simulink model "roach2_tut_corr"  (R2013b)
settings: Solver=VariableStepDiscrete  SolverMode=SingleTasking  StartTime=0.0  StopTime=100  RelTol=1e-3
undefined symbols (not defined in the file): add_latency, addr_width, Bit, bitfield, BitWidth, bram_latency, burst_size, casper_library_scopes, conv_latency, data_width, DelayLen, fan_latency, FFTSize, FFTStage, getfield, increment, led, Location, Lower, mult_latency, mux_latency, n_bits, n_bits_data, n_inputs, n_streams, n_taps, neg_latency, negate_latency, nsamples, pfb_size, pulse_len, reset_period, ROACH, ROACH2, snapshot, sx475t, sync_period, sync_period_bits, Upper, UseCounter, Width
libraries: xbsIndex_r4 x24444, casper_library_misc x73, xbsReplacements_r4 x34, casper_library_delays x14, xps_library x7
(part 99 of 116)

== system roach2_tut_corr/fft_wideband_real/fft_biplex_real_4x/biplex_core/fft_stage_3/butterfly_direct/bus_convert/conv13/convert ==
  note: (ones_bit & 1) -> round-to-even (ones_bit ^ 1) -> round-to-odd (sign_bit & 1)-> round-to-zero (sign_bit ^ 1) -> round-to-inf (X ~| 1) -> round half down (X | 1) -> round half up
  in : Inport
  Concat : xbsIndex_r4/Concat  num_inputs=2  dbl_ovrd=off  block_type=concat
  Constant : xbsIndex_r4/Constant  const=1  gui_display_data_type=Fixed-point  arith_type=Unsigned  n_bits=1  bin_pt=0  preci_type=Single  exp_width=8  frac_width=24  explicit_period=off  period=1  equ=P=C  opselect=C  inp2=PCIN>>17  opr=+  inp1=P  carry=CIN  dbl_ovrd=off  block_type=constant
  Reinterpret : xbsIndex_r4/Reinterpret  force_arith_type=on  arith_type=Unsigned  force_bin_pt=on  bin_pt=0  block_type=reinterpret
  adder : xbsIndex_r4/AddSub  mode=Addition  use_carryin=off  use_carryout=off  en=off  latency=1  precision=User Defined  arith_type="Signed  (2's comp)"  n_bits=18  bin_pt=17  quantization=Truncate  overflow=Wrap  dbl_ovrd=off  use_behavioral_HDL=off  hw_selection=Fabric  pipelined=on  use_rpm=on  block_type=addsub
  almost_half : xbsIndex_r4/Constant  const=1  gui_display_data_type=Fixed-point  arith_type=Unsigned  n_bits=19  bin_pt=0  preci_type=Single  exp_width=8  frac_width=24  explicit_period=off  period=1  equ=P=C  opselect=C  inp2=PCIN>>17  opr=+  inp1=P  carry=CIN  dbl_ovrd=off  block_type=constant
  bit : xbsIndex_r4/Slice  nbits=1  boolean_output=off  mode=Lower Bit Location + Width  bit1=0  base1=MSB of Input  bit0=1  base0=LSB of Input  dbl_ovrd=off  block_type=slice
  force1 : xbsIndex_r4/Reinterpret  force_arith_type=on  arith_type="Signed  (2's comp)"  force_bin_pt=on  bin_pt=19  block_type=reinterpret
  force2 : xbsIndex_r4/Reinterpret  force_arith_type=off  arith_type="Signed  (2's comp)"  force_bin_pt=on  bin_pt=19  block_type=reinterpret
  tweak_op : xbsIndex_r4/Logical  logical_function=AND  inputs=2  en=off  latency=0  precision=Full  arith_type=Unsigned  n_bits=8  bin_pt=2  align_bp=on  dbl_ovrd=off  block_type=logical
  out : Outport
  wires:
  tweak_op/1 -> Concat/2
  Constant/1 -> tweak_op/2
  bit/1 -> tweak_op/1
  almost_half/1 -> force2/1
  in/1 -> Reinterpret/1, bit/1
  Concat/1 -> force1/1
  Reinterpret/1 -> Concat/1
  force1/1 -> adder/1
  force2/1 -> adder/2
  adder/1 -> out/1

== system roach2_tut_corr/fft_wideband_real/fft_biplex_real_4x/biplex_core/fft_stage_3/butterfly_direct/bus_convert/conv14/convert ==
  note: (ones_bit & 1) -> round-to-even (ones_bit ^ 1) -> round-to-odd (sign_bit & 1)-> round-to-zero (sign_bit ^ 1) -> round-to-inf (X ~| 1) -> round half down (X | 1) -> round half up
  in : Inport
  Concat : xbsIndex_r4/Concat  num_inputs=2  dbl_ovrd=off  block_type=concat
  Constant : xbsIndex_r4/Constant  const=1  gui_display_data_type=Fixed-point  arith_type=Unsigned  n_bits=1  bin_pt=0  preci_type=Single  exp_width=8  frac_width=24  explicit_period=off  period=1  equ=P=C  opselect=C  inp2=PCIN>>17  opr=+  inp1=P  carry=CIN  dbl_ovrd=off  block_type=constant
  Reinterpret : xbsIndex_r4/Reinterpret  force_arith_type=on  arith_type=Unsigned  force_bin_pt=on  bin_pt=0  block_type=reinterpret
  adder : xbsIndex_r4/AddSub  mode=Addition  use_carryin=off  use_carryout=off  en=off  latency=1  precision=User Defined  arith_type="Signed  (2's comp)"  n_bits=18  bin_pt=17  quantization=Truncate  overflow=Wrap  dbl_ovrd=off  use_behavioral_HDL=off  hw_selection=Fabric  pipelined=on  use_rpm=on  block_type=addsub
  almost_half : xbsIndex_r4/Constant  const=1  gui_display_data_type=Fixed-point  arith_type=Unsigned  n_bits=19  bin_pt=0  preci_type=Single  exp_width=8  frac_width=24  explicit_period=off  period=1  equ=P=C  opselect=C  inp2=PCIN>>17  opr=+  inp1=P  carry=CIN  dbl_ovrd=off  block_type=constant
  bit : xbsIndex_r4/Slice  nbits=1  boolean_output=off  mode=Lower Bit Location + Width  bit1=0  base1=MSB of Input  bit0=1  base0=LSB of Input  dbl_ovrd=off  block_type=slice
  force1 : xbsIndex_r4/Reinterpret  force_arith_type=on  arith_type="Signed  (2's comp)"  force_bin_pt=on  bin_pt=19  block_type=reinterpret
  force2 : xbsIndex_r4/Reinterpret  force_arith_type=off  arith_type="Signed  (2's comp)"  force_bin_pt=on  bin_pt=19  block_type=reinterpret
  tweak_op : xbsIndex_r4/Logical  logical_function=AND  inputs=2  en=off  latency=0  precision=Full  arith_type=Unsigned  n_bits=8  bin_pt=2  align_bp=on  dbl_ovrd=off  block_type=logical
  out : Outport
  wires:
  tweak_op/1 -> Concat/2
  Constant/1 -> tweak_op/2
  bit/1 -> tweak_op/1
  almost_half/1 -> force2/1
  in/1 -> Reinterpret/1, bit/1
  Concat/1 -> force1/1
  Reinterpret/1 -> Concat/1
  force1/1 -> adder/1
  force2/1 -> adder/2
  adder/1 -> out/1

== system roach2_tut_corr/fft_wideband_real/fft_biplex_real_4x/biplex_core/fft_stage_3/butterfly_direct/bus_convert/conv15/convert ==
  note: (ones_bit & 1) -> round-to-even (ones_bit ^ 1) -> round-to-odd (sign_bit & 1)-> round-to-zero (sign_bit ^ 1) -> round-to-inf (X ~| 1) -> round half down (X | 1) -> round half up
  in : Inport
  Concat : xbsIndex_r4/Concat  num_inputs=2  dbl_ovrd=off  block_type=concat
  Constant : xbsIndex_r4/Constant  const=1  gui_display_data_type=Fixed-point  arith_type=Unsigned  n_bits=1  bin_pt=0  preci_type=Single  exp_width=8  frac_width=24  explicit_period=off  period=1  equ=P=C  opselect=C  inp2=PCIN>>17  opr=+  inp1=P  carry=CIN  dbl_ovrd=off  block_type=constant
  Reinterpret : xbsIndex_r4/Reinterpret  force_arith_type=on  arith_type=Unsigned  force_bin_pt=on  bin_pt=0  block_type=reinterpret
  adder : xbsIndex_r4/AddSub  mode=Addition  use_carryin=off  use_carryout=off  en=off  latency=1  precision=User Defined  arith_type="Signed  (2's comp)"  n_bits=18  bin_pt=17  quantization=Truncate  overflow=Wrap  dbl_ovrd=off  use_behavioral_HDL=off  hw_selection=Fabric  pipelined=on  use_rpm=on  block_type=addsub
  almost_half : xbsIndex_r4/Constant  const=1  gui_display_data_type=Fixed-point  arith_type=Unsigned  n_bits=19  bin_pt=0  preci_type=Single  exp_width=8  frac_width=24  explicit_period=off  period=1  equ=P=C  opselect=C  inp2=PCIN>>17  opr=+  inp1=P  carry=CIN  dbl_ovrd=off  block_type=constant
  bit : xbsIndex_r4/Slice  nbits=1  boolean_output=off  mode=Lower Bit Location + Width  bit1=0  base1=MSB of Input  bit0=1  base0=LSB of Input  dbl_ovrd=off  block_type=slice
  force1 : xbsIndex_r4/Reinterpret  force_arith_type=on  arith_type="Signed  (2's comp)"  force_bin_pt=on  bin_pt=19  block_type=reinterpret
  force2 : xbsIndex_r4/Reinterpret  force_arith_type=off  arith_type="Signed  (2's comp)"  force_bin_pt=on  bin_pt=19  block_type=reinterpret
  tweak_op : xbsIndex_r4/Logical  logical_function=AND  inputs=2  en=off  latency=0  precision=Full  arith_type=Unsigned  n_bits=8  bin_pt=2  align_bp=on  dbl_ovrd=off  block_type=logical
  out : Outport
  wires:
  tweak_op/1 -> Concat/2
  Constant/1 -> tweak_op/2
  bit/1 -> tweak_op/1
  almost_half/1 -> force2/1
  in/1 -> Reinterpret/1, bit/1
  Concat/1 -> force1/1
  Reinterpret/1 -> Concat/1
  force1/1 -> adder/1
  force2/1 -> adder/2
  adder/1 -> out/1

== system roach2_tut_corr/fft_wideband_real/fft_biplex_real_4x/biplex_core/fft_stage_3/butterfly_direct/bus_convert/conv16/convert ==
  note: (ones_bit & 1) -> round-to-even (ones_bit ^ 1) -> round-to-odd (sign_bit & 1)-> round-to-zero (sign_bit ^ 1) -> round-to-inf (X ~| 1) -> round half down (X | 1) -> round half up
  in : Inport
  Concat : xbsIndex_r4/Concat  num_inputs=2  dbl_ovrd=off  block_type=concat
  Constant : xbsIndex_r4/Constant  const=1  gui_display_data_type=Fixed-point  arith_type=Unsigned  n_bits=1  bin_pt=0  preci_type=Single  exp_width=8  frac_width=24  explicit_period=off  period=1  equ=P=C  opselect=C  inp2=PCIN>>17  opr=+  inp1=P  carry=CIN  dbl_ovrd=off  block_type=constant
  Reinterpret : xbsIndex_r4/Reinterpret  force_arith_type=on  arith_type=Unsigned  force_bin_pt=on  bin_pt=0  block_type=reinterpret
  adder : xbsIndex_r4/AddSub  mode=Addition  use_carryin=off  use_carryout=off  en=off  latency=1  precision=User Defined  arith_type="Signed  (2's comp)"  n_bits=18  bin_pt=17  quantization=Truncate  overflow=Wrap  dbl_ovrd=off  use_behavioral_HDL=off  hw_selection=Fabric  pipelined=on  use_rpm=on  block_type=addsub
  almost_half : xbsIndex_r4/Constant  const=1  gui_display_data_type=Fixed-point  arith_type=Unsigned  n_bits=19  bin_pt=0  preci_type=Single  exp_width=8  frac_width=24  explicit_period=off  period=1  equ=P=C  opselect=C  inp2=PCIN>>17  opr=+  inp1=P  carry=CIN  dbl_ovrd=off  block_type=constant
  bit : xbsIndex_r4/Slice  nbits=1  boolean_output=off  mode=Lower Bit Location + Width  bit1=0  base1=MSB of Input  bit0=1  base0=LSB of Input  dbl_ovrd=off  block_type=slice
  force1 : xbsIndex_r4/Reinterpret  force_arith_type=on  arith_type="Signed  (2's comp)"  force_bin_pt=on  bin_pt=19  block_type=reinterpret
  force2 : xbsIndex_r4/Reinterpret  force_arith_type=off  arith_type="Signed  (2's comp)"  force_bin_pt=on  bin_pt=19  block_type=reinterpret
  tweak_op : xbsIndex_r4/Logical  logical_function=AND  inputs=2  en=off  latency=0  precision=Full  arith_type=Unsigned  n_bits=8  bin_pt=2  align_bp=on  dbl_ovrd=off  block_type=logical
  out : Outport
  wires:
  tweak_op/1 -> Concat/2
  Constant/1 -> tweak_op/2
  bit/1 -> tweak_op/1
  almost_half/1 -> force2/1
  in/1 -> Reinterpret/1, bit/1
  Concat/1 -> force1/1
  Reinterpret/1 -> Concat/1
  force1/1 -> adder/1
  force2/1 -> adder/2
  adder/1 -> out/1

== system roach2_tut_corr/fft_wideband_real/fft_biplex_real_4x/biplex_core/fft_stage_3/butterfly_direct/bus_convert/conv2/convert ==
  note: (ones_bit & 1) -> round-to-even (ones_bit ^ 1) -> round-to-odd (sign_bit & 1)-> round-to-zero (sign_bit ^ 1) -> round-to-inf (X ~| 1) -> round half down (X | 1) -> round half up
  in : Inport
  Concat : xbsIndex_r4/Concat  num_inputs=2  dbl_ovrd=off  block_type=concat
  Constant : xbsIndex_r4/Constant  const=1  gui_display_data_type=Fixed-point  arith_type=Unsigned  n_bits=1  bin_pt=0  preci_type=Single  exp_width=8  frac_width=24  explicit_period=off  period=1  equ=P=C  opselect=C  inp2=PCIN>>17  opr=+  inp1=P  carry=CIN  dbl_ovrd=off  block_type=constant
  Reinterpret : xbsIndex_r4/Reinterpret  force_arith_type=on  arith_type=Unsigned  force_bin_pt=on  bin_pt=0  block_type=reinterpret
  adder : xbsIndex_r4/AddSub  mode=Addition  use_carryin=off  use_carryout=off  en=off  latency=1  precision=User Defined  arith_type="Signed  (2's comp)"  n_bits=18  bin_pt=17  quantization=Truncate  overflow=Wrap  dbl_ovrd=off  use_behavioral_HDL=off  hw_selection=Fabric  pipelined=on  use_rpm=on  block_type=addsub
  almost_half : xbsIndex_r4/Constant  const=1  gui_display_data_type=Fixed-point  arith_type=Unsigned  n_bits=19  bin_pt=0  preci_type=Single  exp_width=8  frac_width=24  explicit_period=off  period=1  equ=P=C  opselect=C  inp2=PCIN>>17  opr=+  inp1=P  carry=CIN  dbl_ovrd=off  block_type=constant
  bit : xbsIndex_r4/Slice  nbits=1  boolean_output=off  mode=Lower Bit Location + Width  bit1=0  base1=MSB of Input  bit0=1  base0=LSB of Input  dbl_ovrd=off  block_type=slice
  force1 : xbsIndex_r4/Reinterpret  force_arith_type=on  arith_type="Signed  (2's comp)"  force_bin_pt=on  bin_pt=19  block_type=reinterpret
  force2 : xbsIndex_r4/Reinterpret  force_arith_type=off  arith_type="Signed  (2's comp)"  force_bin_pt=on  bin_pt=19  block_type=reinterpret
  tweak_op : xbsIndex_r4/Logical  logical_function=AND  inputs=2  en=off  latency=0  precision=Full  arith_type=Unsigned  n_bits=8  bin_pt=2  align_bp=on  dbl_ovrd=off  block_type=logical
  out : Outport
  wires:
  tweak_op/1 -> Concat/2
  Constant/1 -> tweak_op/2
  bit/1 -> tweak_op/1
  almost_half/1 -> force2/1
  in/1 -> Reinterpret/1, bit/1
  Concat/1 -> force1/1
  Reinterpret/1 -> Concat/1
  force1/1 -> adder/1
  force2/1 -> adder/2
  adder/1 -> out/1

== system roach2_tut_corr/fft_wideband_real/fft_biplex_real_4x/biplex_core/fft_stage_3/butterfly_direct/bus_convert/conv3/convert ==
  note: (ones_bit & 1) -> round-to-even (ones_bit ^ 1) -> round-to-odd (sign_bit & 1)-> round-to-zero (sign_bit ^ 1) -> round-to-inf (X ~| 1) -> round half down (X | 1) -> round half up
  in : Inport
  Concat : xbsIndex_r4/Concat  num_inputs=2  dbl_ovrd=off  block_type=concat
  Constant : xbsIndex_r4/Constant  const=1  gui_display_data_type=Fixed-point  arith_type=Unsigned  n_bits=1  bin_pt=0  preci_type=Single  exp_width=8  frac_width=24  explicit_period=off  period=1  equ=P=C  opselect=C  inp2=PCIN>>17  opr=+  inp1=P  carry=CIN  dbl_ovrd=off  block_type=constant
  Reinterpret : xbsIndex_r4/Reinterpret  force_arith_type=on  arith_type=Unsigned  force_bin_pt=on  bin_pt=0  block_type=reinterpret
  adder : xbsIndex_r4/AddSub  mode=Addition  use_carryin=off  use_carryout=off  en=off  latency=1  precision=User Defined  arith_type="Signed  (2's comp)"  n_bits=18  bin_pt=17  quantization=Truncate  overflow=Wrap  dbl_ovrd=off  use_behavioral_HDL=off  hw_selection=Fabric  pipelined=on  use_rpm=on  block_type=addsub
  almost_half : xbsIndex_r4/Constant  const=1  gui_display_data_type=Fixed-point  arith_type=Unsigned  n_bits=19  bin_pt=0  preci_type=Single  exp_width=8  frac_width=24  explicit_period=off  period=1  equ=P=C  opselect=C  inp2=PCIN>>17  opr=+  inp1=P  carry=CIN  dbl_ovrd=off  block_type=constant
  bit : xbsIndex_r4/Slice  nbits=1  boolean_output=off  mode=Lower Bit Location + Width  bit1=0  base1=MSB of Input  bit0=1  base0=LSB of Input  dbl_ovrd=off  block_type=slice
  force1 : xbsIndex_r4/Reinterpret  force_arith_type=on  arith_type="Signed  (2's comp)"  force_bin_pt=on  bin_pt=19  block_type=reinterpret
  force2 : xbsIndex_r4/Reinterpret  force_arith_type=off  arith_type="Signed  (2's comp)"  force_bin_pt=on  bin_pt=19  block_type=reinterpret
  tweak_op : xbsIndex_r4/Logical  logical_function=AND  inputs=2  en=off  latency=0  precision=Full  arith_type=Unsigned  n_bits=8  bin_pt=2  align_bp=on  dbl_ovrd=off  block_type=logical
  out : Outport
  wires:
  tweak_op/1 -> Concat/2
  Constant/1 -> tweak_op/2
  bit/1 -> tweak_op/1
  almost_half/1 -> force2/1
  in/1 -> Reinterpret/1, bit/1
  Concat/1 -> force1/1
  Reinterpret/1 -> Concat/1
  force1/1 -> adder/1
  force2/1 -> adder/2
  adder/1 -> out/1

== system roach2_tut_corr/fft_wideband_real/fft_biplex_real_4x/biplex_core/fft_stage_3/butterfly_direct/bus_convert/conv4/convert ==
  note: (ones_bit & 1) -> round-to-even (ones_bit ^ 1) -> round-to-odd (sign_bit & 1)-> round-to-zero (sign_bit ^ 1) -> round-to-inf (X ~| 1) -> round half down (X | 1) -> round half up
  in : Inport
  Concat : xbsIndex_r4/Concat  num_inputs=2  dbl_ovrd=off  block_type=concat
  Constant : xbsIndex_r4/Constant  const=1  gui_display_data_type=Fixed-point  arith_type=Unsigned  n_bits=1  bin_pt=0  preci_type=Single  exp_width=8  frac_width=24  explicit_period=off  period=1  equ=P=C  opselect=C  inp2=PCIN>>17  opr=+  inp1=P  carry=CIN  dbl_ovrd=off  block_type=constant
  Reinterpret : xbsIndex_r4/Reinterpret  force_arith_type=on  arith_type=Unsigned  force_bin_pt=on  bin_pt=0  block_type=reinterpret
  adder : xbsIndex_r4/AddSub  mode=Addition  use_carryin=off  use_carryout=off  en=off  latency=1  precision=User Defined  arith_type="Signed  (2's comp)"  n_bits=18  bin_pt=17  quantization=Truncate  overflow=Wrap  dbl_ovrd=off  use_behavioral_HDL=off  hw_selection=Fabric  pipelined=on  use_rpm=on  block_type=addsub
  almost_half : xbsIndex_r4/Constant  const=1  gui_display_data_type=Fixed-point  arith_type=Unsigned  n_bits=19  bin_pt=0  preci_type=Single  exp_width=8  frac_width=24  explicit_period=off  period=1  equ=P=C  opselect=C  inp2=PCIN>>17  opr=+  inp1=P  carry=CIN  dbl_ovrd=off  block_type=constant
  bit : xbsIndex_r4/Slice  nbits=1  boolean_output=off  mode=Lower Bit Location + Width  bit1=0  base1=MSB of Input  bit0=1  base0=LSB of Input  dbl_ovrd=off  block_type=slice
  force1 : xbsIndex_r4/Reinterpret  force_arith_type=on  arith_type="Signed  (2's comp)"  force_bin_pt=on  bin_pt=19  block_type=reinterpret
  force2 : xbsIndex_r4/Reinterpret  force_arith_type=off  arith_type="Signed  (2's comp)"  force_bin_pt=on  bin_pt=19  block_type=reinterpret
  tweak_op : xbsIndex_r4/Logical  logical_function=AND  inputs=2  en=off  latency=0  precision=Full  arith_type=Unsigned  n_bits=8  bin_pt=2  align_bp=on  dbl_ovrd=off  block_type=logical
  out : Outport
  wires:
  tweak_op/1 -> Concat/2
  Constant/1 -> tweak_op/2
  bit/1 -> tweak_op/1
  almost_half/1 -> force2/1
  in/1 -> Reinterpret/1, bit/1
  Concat/1 -> force1/1
  Reinterpret/1 -> Concat/1
  force1/1 -> adder/1
  force2/1 -> adder/2
  adder/1 -> out/1

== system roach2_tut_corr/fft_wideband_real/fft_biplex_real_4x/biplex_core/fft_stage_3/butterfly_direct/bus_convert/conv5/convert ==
  note: (ones_bit & 1) -> round-to-even (ones_bit ^ 1) -> round-to-odd (sign_bit & 1)-> round-to-zero (sign_bit ^ 1) -> round-to-inf (X ~| 1) -> round half down (X | 1) -> round half up
  in : Inport
  Concat : xbsIndex_r4/Concat  num_inputs=2  dbl_ovrd=off  block_type=concat
  Constant : xbsIndex_r4/Constant  const=1  gui_display_data_type=Fixed-point  arith_type=Unsigned  n_bits=1  bin_pt=0  preci_type=Single  exp_width=8  frac_width=24  explicit_period=off  period=1  equ=P=C  opselect=C  inp2=PCIN>>17  opr=+  inp1=P  carry=CIN  dbl_ovrd=off  block_type=constant
  Reinterpret : xbsIndex_r4/Reinterpret  force_arith_type=on  arith_type=Unsigned  force_bin_pt=on  bin_pt=0  block_type=reinterpret
  adder : xbsIndex_r4/AddSub  mode=Addition  use_carryin=off  use_carryout=off  en=off  latency=1  precision=User Defined  arith_type="Signed  (2's comp)"  n_bits=18  bin_pt=17  quantization=Truncate  overflow=Wrap  dbl_ovrd=off  use_behavioral_HDL=off  hw_selection=Fabric  pipelined=on  use_rpm=on  block_type=addsub
  almost_half : xbsIndex_r4/Constant  const=1  gui_display_data_type=Fixed-point  arith_type=Unsigned  n_bits=19  bin_pt=0  preci_type=Single  exp_width=8  frac_width=24  explicit_period=off  period=1  equ=P=C  opselect=C  inp2=PCIN>>17  opr=+  inp1=P  carry=CIN  dbl_ovrd=off  block_type=constant
  bit : xbsIndex_r4/Slice  nbits=1  boolean_output=off  mode=Lower Bit Location + Width  bit1=0  base1=MSB of Input  bit0=1  base0=LSB of Input  dbl_ovrd=off  block_type=slice
  force1 : xbsIndex_r4/Reinterpret  force_arith_type=on  arith_type="Signed  (2's comp)"  force_bin_pt=on  bin_pt=19  block_type=reinterpret
  force2 : xbsIndex_r4/Reinterpret  force_arith_type=off  arith_type="Signed  (2's comp)"  force_bin_pt=on  bin_pt=19  block_type=reinterpret
  tweak_op : xbsIndex_r4/Logical  logical_function=AND  inputs=2  en=off  latency=0  precision=Full  arith_type=Unsigned  n_bits=8  bin_pt=2  align_bp=on  dbl_ovrd=off  block_type=logical
  out : Outport
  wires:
  tweak_op/1 -> Concat/2
  Constant/1 -> tweak_op/2
  bit/1 -> tweak_op/1
  almost_half/1 -> force2/1
  in/1 -> Reinterpret/1, bit/1
  Concat/1 -> force1/1
  Reinterpret/1 -> Concat/1
  force1/1 -> adder/1
  force2/1 -> adder/2
  adder/1 -> out/1

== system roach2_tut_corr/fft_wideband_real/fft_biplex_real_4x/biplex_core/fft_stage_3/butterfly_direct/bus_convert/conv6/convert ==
  note: (ones_bit & 1) -> round-to-even (ones_bit ^ 1) -> round-to-odd (sign_bit & 1)-> round-to-zero (sign_bit ^ 1) -> round-to-inf (X ~| 1) -> round half down (X | 1) -> round half up
  in : Inport
  Concat : xbsIndex_r4/Concat  num_inputs=2  dbl_ovrd=off  block_type=concat
  Constant : xbsIndex_r4/Constant  const=1  gui_display_data_type=Fixed-point  arith_type=Unsigned  n_bits=1  bin_pt=0  preci_type=Single  exp_width=8  frac_width=24  explicit_period=off  period=1  equ=P=C  opselect=C  inp2=PCIN>>17  opr=+  inp1=P  carry=CIN  dbl_ovrd=off  block_type=constant
  Reinterpret : xbsIndex_r4/Reinterpret  force_arith_type=on  arith_type=Unsigned  force_bin_pt=on  bin_pt=0  block_type=reinterpret
  adder : xbsIndex_r4/AddSub  mode=Addition  use_carryin=off  use_carryout=off  en=off  latency=1  precision=User Defined  arith_type="Signed  (2's comp)"  n_bits=18  bin_pt=17  quantization=Truncate  overflow=Wrap  dbl_ovrd=off  use_behavioral_HDL=off  hw_selection=Fabric  pipelined=on  use_rpm=on  block_type=addsub
  almost_half : xbsIndex_r4/Constant  const=1  gui_display_data_type=Fixed-point  arith_type=Unsigned  n_bits=19  bin_pt=0  preci_type=Single  exp_width=8  frac_width=24  explicit_period=off  period=1  equ=P=C  opselect=C  inp2=PCIN>>17  opr=+  inp1=P  carry=CIN  dbl_ovrd=off  block_type=constant
  bit : xbsIndex_r4/Slice  nbits=1  boolean_output=off  mode=Lower Bit Location + Width  bit1=0  base1=MSB of Input  bit0=1  base0=LSB of Input  dbl_ovrd=off  block_type=slice
  force1 : xbsIndex_r4/Reinterpret  force_arith_type=on  arith_type="Signed  (2's comp)"  force_bin_pt=on  bin_pt=19  block_type=reinterpret
  force2 : xbsIndex_r4/Reinterpret  force_arith_type=off  arith_type="Signed  (2's comp)"  force_bin_pt=on  bin_pt=19  block_type=reinterpret
  tweak_op : xbsIndex_r4/Logical  logical_function=AND  inputs=2  en=off  latency=0  precision=Full  arith_type=Unsigned  n_bits=8  bin_pt=2  align_bp=on  dbl_ovrd=off  block_type=logical
  out : Outport
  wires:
  tweak_op/1 -> Concat/2
  Constant/1 -> tweak_op/2
  bit/1 -> tweak_op/1
  almost_half/1 -> force2/1
  in/1 -> Reinterpret/1, bit/1
  Concat/1 -> force1/1
  Reinterpret/1 -> Concat/1
  force1/1 -> adder/1
  force2/1 -> adder/2
  adder/1 -> out/1

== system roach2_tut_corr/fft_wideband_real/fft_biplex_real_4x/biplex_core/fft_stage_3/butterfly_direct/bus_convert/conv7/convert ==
  note: (ones_bit & 1) -> round-to-even (ones_bit ^ 1) -> round-to-odd (sign_bit & 1)-> round-to-zero (sign_bit ^ 1) -> round-to-inf (X ~| 1) -> round half down (X | 1) -> round half up
  in : Inport
  Concat : xbsIndex_r4/Concat  num_inputs=2  dbl_ovrd=off  block_type=concat
  Constant : xbsIndex_r4/Constant  const=1  gui_display_data_type=Fixed-point  arith_type=Unsigned  n_bits=1  bin_pt=0  preci_type=Single  exp_width=8  frac_width=24  explicit_period=off  period=1  equ=P=C  opselect=C  inp2=PCIN>>17  opr=+  inp1=P  carry=CIN  dbl_ovrd=off  block_type=constant
  Reinterpret : xbsIndex_r4/Reinterpret  force_arith_type=on  arith_type=Unsigned  force_bin_pt=on  bin_pt=0  block_type=reinterpret
  adder : xbsIndex_r4/AddSub  mode=Addition  use_carryin=off  use_carryout=off  en=off  latency=1  precision=User Defined  arith_type="Signed  (2's comp)"  n_bits=18  bin_pt=17  quantization=Truncate  overflow=Wrap  dbl_ovrd=off  use_behavioral_HDL=off  hw_selection=Fabric  pipelined=on  use_rpm=on  block_type=addsub
  almost_half : xbsIndex_r4/Constant  const=1  gui_display_data_type=Fixed-point  arith_type=Unsigned  n_bits=19  bin_pt=0  preci_type=Single  exp_width=8  frac_width=24  explicit_period=off  period=1  equ=P=C  opselect=C  inp2=PCIN>>17  opr=+  inp1=P  carry=CIN  dbl_ovrd=off  block_type=constant
  bit : xbsIndex_r4/Slice  nbits=1  boolean_output=off  mode=Lower Bit Location + Width  bit1=0  base1=MSB of Input  bit0=1  base0=LSB of Input  dbl_ovrd=off  block_type=slice
  force1 : xbsIndex_r4/Reinterpret  force_arith_type=on  arith_type="Signed  (2's comp)"  force_bin_pt=on  bin_pt=19  block_type=reinterpret
  force2 : xbsIndex_r4/Reinterpret  force_arith_type=off  arith_type="Signed  (2's comp)"  force_bin_pt=on  bin_pt=19  block_type=reinterpret
  tweak_op : xbsIndex_r4/Logical  logical_function=AND  inputs=2  en=off  latency=0  precision=Full  arith_type=Unsigned  n_bits=8  bin_pt=2  align_bp=on  dbl_ovrd=off  block_type=logical
  out : Outport
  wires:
  tweak_op/1 -> Concat/2
  Constant/1 -> tweak_op/2
  bit/1 -> tweak_op/1
  almost_half/1 -> force2/1
  in/1 -> Reinterpret/1, bit/1
  Concat/1 -> force1/1
  Reinterpret/1 -> Concat/1
  force1/1 -> adder/1
  force2/1 -> adder/2
  adder/1 -> out/1

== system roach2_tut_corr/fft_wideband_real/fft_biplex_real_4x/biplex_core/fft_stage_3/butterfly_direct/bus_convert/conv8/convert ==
  note: (ones_bit & 1) -> round-to-even (ones_bit ^ 1) -> round-to-odd (sign_bit & 1)-> round-to-zero (sign_bit ^ 1) -> round-to-inf (X ~| 1) -> round half down (X | 1) -> round half up
  in : Inport
  Concat : xbsIndex_r4/Concat  num_inputs=2  dbl_ovrd=off  block_type=concat
  Constant : xbsIndex_r4/Constant  const=1  gui_display_data_type=Fixed-point  arith_type=Unsigned  n_bits=1  bin_pt=0  preci_type=Single  exp_width=8  frac_width=24  explicit_period=off  period=1  equ=P=C  opselect=C  inp2=PCIN>>17  opr=+  inp1=P  carry=CIN  dbl_ovrd=off  block_type=constant
  Reinterpret : xbsIndex_r4/Reinterpret  force_arith_type=on  arith_type=Unsigned  force_bin_pt=on  bin_pt=0  block_type=reinterpret
  adder : xbsIndex_r4/AddSub  mode=Addition  use_carryin=off  use_carryout=off  en=off  latency=1  precision=User Defined  arith_type="Signed  (2's comp)"  n_bits=18  bin_pt=17  quantization=Truncate  overflow=Wrap  dbl_ovrd=off  use_behavioral_HDL=off  hw_selection=Fabric  pipelined=on  use_rpm=on  block_type=addsub
  almost_half : xbsIndex_r4/Constant  const=1  gui_display_data_type=Fixed-point  arith_type=Unsigned  n_bits=19  bin_pt=0  preci_type=Single  exp_width=8  frac_width=24  explicit_period=off  period=1  equ=P=C  opselect=C  inp2=PCIN>>17  opr=+  inp1=P  carry=CIN  dbl_ovrd=off  block_type=constant
  bit : xbsIndex_r4/Slice  nbits=1  boolean_output=off  mode=Lower Bit Location + Width  bit1=0  base1=MSB of Input  bit0=1  base0=LSB of Input  dbl_ovrd=off  block_type=slice
  force1 : xbsIndex_r4/Reinterpret  force_arith_type=on  arith_type="Signed  (2's comp)"  force_bin_pt=on  bin_pt=19  block_type=reinterpret
  force2 : xbsIndex_r4/Reinterpret  force_arith_type=off  arith_type="Signed  (2's comp)"  force_bin_pt=on  bin_pt=19  block_type=reinterpret
  tweak_op : xbsIndex_r4/Logical  logical_function=AND  inputs=2  en=off  latency=0  precision=Full  arith_type=Unsigned  n_bits=8  bin_pt=2  align_bp=on  dbl_ovrd=off  block_type=logical
  out : Outport
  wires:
  tweak_op/1 -> Concat/2
  Constant/1 -> tweak_op/2
  bit/1 -> tweak_op/1
  almost_half/1 -> force2/1
  in/1 -> Reinterpret/1, bit/1
  Concat/1 -> force1/1
  Reinterpret/1 -> Concat/1
  force1/1 -> adder/1
  force2/1 -> adder/2
  adder/1 -> out/1

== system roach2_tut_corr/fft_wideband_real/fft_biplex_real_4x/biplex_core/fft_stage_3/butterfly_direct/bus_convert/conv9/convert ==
  note: (ones_bit & 1) -> round-to-even (ones_bit ^ 1) -> round-to-odd (sign_bit & 1)-> round-to-zero (sign_bit ^ 1) -> round-to-inf (X ~| 1) -> round half down (X | 1) -> round half up
  in : Inport
  Concat : xbsIndex_r4/Concat  num_inputs=2  dbl_ovrd=off  block_type=concat
  Constant : xbsIndex_r4/Constant  const=1  gui_display_data_type=Fixed-point  arith_type=Unsigned  n_bits=1  bin_pt=0  preci_type=Single  exp_width=8  frac_width=24  explicit_period=off  period=1  equ=P=C  opselect=C  inp2=PCIN>>17  opr=+  inp1=P  carry=CIN  dbl_ovrd=off  block_type=constant
  Reinterpret : xbsIndex_r4/Reinterpret  force_arith_type=on  arith_type=Unsigned  force_bin_pt=on  bin_pt=0  block_type=reinterpret
  adder : xbsIndex_r4/AddSub  mode=Addition  use_carryin=off  use_carryout=off  en=off  latency=1  precision=User Defined  arith_type="Signed  (2's comp)"  n_bits=18  bin_pt=17  quantization=Truncate  overflow=Wrap  dbl_ovrd=off  use_behavioral_HDL=off  hw_selection=Fabric  pipelined=on  use_rpm=on  block_type=addsub
  almost_half : xbsIndex_r4/Constant  const=1  gui_display_data_type=Fixed-point  arith_type=Unsigned  n_bits=19  bin_pt=0  preci_type=Single  exp_width=8  frac_width=24  explicit_period=off  period=1  equ=P=C  opselect=C  inp2=PCIN>>17  opr=+  inp1=P  carry=CIN  dbl_ovrd=off  block_type=constant
  bit : xbsIndex_r4/Slice  nbits=1  boolean_output=off  mode=Lower Bit Location + Width  bit1=0  base1=MSB of Input  bit0=1  base0=LSB of Input  dbl_ovrd=off  block_type=slice
  force1 : xbsIndex_r4/Reinterpret  force_arith_type=on  arith_type="Signed  (2's comp)"  force_bin_pt=on  bin_pt=19  block_type=reinterpret
  force2 : xbsIndex_r4/Reinterpret  force_arith_type=off  arith_type="Signed  (2's comp)"  force_bin_pt=on  bin_pt=19  block_type=reinterpret
  tweak_op : xbsIndex_r4/Logical  logical_function=AND  inputs=2  en=off  latency=0  precision=Full  arith_type=Unsigned  n_bits=8  bin_pt=2  align_bp=on  dbl_ovrd=off  block_type=logical
  out : Outport
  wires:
  tweak_op/1 -> Concat/2
  Constant/1 -> tweak_op/2
  bit/1 -> tweak_op/1
  almost_half/1 -> force2/1
  in/1 -> Reinterpret/1, bit/1
  Concat/1 -> force1/1
  Reinterpret/1 -> Concat/1
  force1/1 -> adder/1
  force2/1 -> adder/2
  adder/1 -> out/1

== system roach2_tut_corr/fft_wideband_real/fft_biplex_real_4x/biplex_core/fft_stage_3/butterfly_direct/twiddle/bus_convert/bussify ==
  in1 : Inport
  in2 : Inport  Port=2
  in3 : Inport  Port=3
  in4 : Inport  Port=4
  in5 : Inport  Port=5
  in6 : Inport  Port=6
  in7 : Inport  Port=7
  in8 : Inport  Port=8
  concatenate : xbsIndex_r4/Concat  num_inputs=8  dbl_ovrd=off  block_type=concat
  reinterpret{1..8} (8 alike) : xbsIndex_r4/Reinterpret  force_arith_type=on  arith_type=Unsigned  force_bin_pt=on  bin_pt=0  block_type=reinterpret
  bus_out : Outport
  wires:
  concatenate/1 -> bus_out/1
  in1/1 -> reinterpret1/1
  reinterpret1/1 -> concatenate/1
  in2/1 -> reinterpret2/1
  reinterpret2/1 -> concatenate/2
  in3/1 -> reinterpret3/1
  reinterpret3/1 -> concatenate/3
  in4/1 -> reinterpret4/1
  reinterpret4/1 -> concatenate/4
  in5/1 -> reinterpret5/1
  reinterpret5/1 -> concatenate/5
  in6/1 -> reinterpret6/1
  reinterpret6/1 -> concatenate/6
  in7/1 -> reinterpret7/1
  reinterpret7/1 -> concatenate/7
  in8/1 -> reinterpret8/1
  reinterpret8/1 -> concatenate/8

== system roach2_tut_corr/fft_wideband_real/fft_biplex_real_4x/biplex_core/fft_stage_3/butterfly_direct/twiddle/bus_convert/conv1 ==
  note: (ones_bit & 1) -> round-to-even (ones_bit ^ 1) -> round-to-odd (sign_bit & 1)-> round-to-zero (sign_bit ^ 1) -> round-to-inf (X ~| 1) -> round half down (X | 1) -> round half up
  in : Inport
  Concat : xbsIndex_r4/Concat  num_inputs=2  dbl_ovrd=off  block_type=concat
  Constant : xbsIndex_r4/Constant  const=1  gui_display_data_type=Fixed-point  arith_type=Unsigned  n_bits=1  bin_pt=0  preci_type=Single  exp_width=8  frac_width=24  explicit_period=off  period=1  equ=P=C  opselect=C  inp2=PCIN>>17  opr=+  inp1=P  carry=CIN  dbl_ovrd=off  block_type=constant
  Reinterpret : xbsIndex_r4/Reinterpret  force_arith_type=on  arith_type=Unsigned  force_bin_pt=on  bin_pt=0  block_type=reinterpret
  adder : xbsIndex_r4/AddSub  mode=Addition  use_carryin=off  use_carryout=off  en=off  latency=1  precision=User Defined  arith_type="Signed  (2's comp)"  n_bits=19  bin_pt=17  quantization=Truncate  overflow=Wrap  dbl_ovrd=off  use_behavioral_HDL=off  hw_selection=Fabric  pipelined=on  use_rpm=on  block_type=addsub
  almost_half : xbsIndex_r4/Constant  const=131071  gui_display_data_type=Fixed-point  arith_type=Unsigned  n_bits=35  bin_pt=0  preci_type=Single  exp_width=8  frac_width=24  explicit_period=off  period=1  equ=P=C  opselect=C  inp2=PCIN>>17  opr=+  inp1=P  carry=CIN  dbl_ovrd=off  block_type=constant
  bit : xbsIndex_r4/Slice  nbits=1  boolean_output=off  mode=Lower Bit Location + Width  bit1=0  base1=MSB of Input  bit0=17  base0=LSB of Input  dbl_ovrd=off  block_type=slice
  force1 : xbsIndex_r4/Reinterpret  force_arith_type=on  arith_type="Signed  (2's comp)"  force_bin_pt=on  bin_pt=35  block_type=reinterpret
  force2 : xbsIndex_r4/Reinterpret  force_arith_type=off  arith_type="Signed  (2's comp)"  force_bin_pt=on  bin_pt=35  block_type=reinterpret
  tweak_op : xbsIndex_r4/Logical  logical_function=AND  inputs=2  en=off  latency=0  precision=Full  arith_type=Unsigned  n_bits=8  bin_pt=2  align_bp=on  dbl_ovrd=off  block_type=logical
  out : Outport
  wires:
  tweak_op/1 -> Concat/2
  Constant/1 -> tweak_op/2
  bit/1 -> tweak_op/1
  almost_half/1 -> force2/1
  in/1 -> Reinterpret/1, bit/1
  Concat/1 -> force1/1
  Reinterpret/1 -> Concat/1
  force1/1 -> adder/1
  force2/1 -> adder/2
  adder/1 -> out/1

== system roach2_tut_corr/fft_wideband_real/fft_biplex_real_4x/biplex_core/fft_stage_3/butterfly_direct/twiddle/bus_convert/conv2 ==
  note: (ones_bit & 1) -> round-to-even (ones_bit ^ 1) -> round-to-odd (sign_bit & 1)-> round-to-zero (sign_bit ^ 1) -> round-to-inf (X ~| 1) -> round half down (X | 1) -> round half up
  in : Inport
  Concat : xbsIndex_r4/Concat  num_inputs=2  dbl_ovrd=off  block_type=concat
  Constant : xbsIndex_r4/Constant  const=1  gui_display_data_type=Fixed-point  arith_type=Unsigned  n_bits=1  bin_pt=0  preci_type=Single  exp_width=8  frac_width=24  explicit_period=off  period=1  equ=P=C  opselect=C  inp2=PCIN>>17  opr=+  inp1=P  carry=CIN  dbl_ovrd=off  block_type=constant
  Reinterpret : xbsIndex_r4/Reinterpret  force_arith_type=on  arith_type=Unsigned  force_bin_pt=on  bin_pt=0  block_type=reinterpret
  adder : xbsIndex_r4/AddSub  mode=Addition  use_carryin=off  use_carryout=off  en=off  latency=1  precision=User Defined  arith_type="Signed  (2's comp)"  n_bits=19  bin_pt=17  quantization=Truncate  overflow=Wrap  dbl_ovrd=off  use_behavioral_HDL=off  hw_selection=Fabric  pipelined=on  use_rpm=on  block_type=addsub
  almost_half : xbsIndex_r4/Constant  const=131071  gui_display_data_type=Fixed-point  arith_type=Unsigned  n_bits=35  bin_pt=0  preci_type=Single  exp_width=8  frac_width=24  explicit_period=off  period=1  equ=P=C  opselect=C  inp2=PCIN>>17  opr=+  inp1=P  carry=CIN  dbl_ovrd=off  block_type=constant
  bit : xbsIndex_r4/Slice  nbits=1  boolean_output=off  mode=Lower Bit Location + Width  bit1=0  base1=MSB of Input  bit0=17  base0=LSB of Input  dbl_ovrd=off  block_type=slice
  force1 : xbsIndex_r4/Reinterpret  force_arith_type=on  arith_type="Signed  (2's comp)"  force_bin_pt=on  bin_pt=35  block_type=reinterpret
  force2 : xbsIndex_r4/Reinterpret  force_arith_type=off  arith_type="Signed  (2's comp)"  force_bin_pt=on  bin_pt=35  block_type=reinterpret
  tweak_op : xbsIndex_r4/Logical  logical_function=AND  inputs=2  en=off  latency=0  precision=Full  arith_type=Unsigned  n_bits=8  bin_pt=2  align_bp=on  dbl_ovrd=off  block_type=logical
  out : Outport
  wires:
  tweak_op/1 -> Concat/2
  Constant/1 -> tweak_op/2
  bit/1 -> tweak_op/1
  almost_half/1 -> force2/1
  in/1 -> Reinterpret/1, bit/1
  Concat/1 -> force1/1
  Reinterpret/1 -> Concat/1
  force1/1 -> adder/1
  force2/1 -> adder/2
  adder/1 -> out/1

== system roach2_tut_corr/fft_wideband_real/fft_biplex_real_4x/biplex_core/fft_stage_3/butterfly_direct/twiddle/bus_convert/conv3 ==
  note: (ones_bit & 1) -> round-to-even (ones_bit ^ 1) -> round-to-odd (sign_bit & 1)-> round-to-zero (sign_bit ^ 1) -> round-to-inf (X ~| 1) -> round half down (X | 1) -> round half up
  in : Inport
  Concat : xbsIndex_r4/Concat  num_inputs=2  dbl_ovrd=off  block_type=concat
  Constant : xbsIndex_r4/Constant  const=1  gui_display_data_type=Fixed-point  arith_type=Unsigned  n_bits=1  bin_pt=0  preci_type=Single  exp_width=8  frac_width=24  explicit_period=off  period=1  equ=P=C  opselect=C  inp2=PCIN>>17  opr=+  inp1=P  carry=CIN  dbl_ovrd=off  block_type=constant
  Reinterpret : xbsIndex_r4/Reinterpret  force_arith_type=on  arith_type=Unsigned  force_bin_pt=on  bin_pt=0  block_type=reinterpret
  adder : xbsIndex_r4/AddSub  mode=Addition  use_carryin=off  use_carryout=off  en=off  latency=1  precision=User Defined  arith_type="Signed  (2's comp)"  n_bits=19  bin_pt=17  quantization=Truncate  overflow=Wrap  dbl_ovrd=off  use_behavioral_HDL=off  hw_selection=Fabric  pipelined=on  use_rpm=on  block_type=addsub
  almost_half : xbsIndex_r4/Constant  const=131071  gui_display_data_type=Fixed-point  arith_type=Unsigned  n_bits=35  bin_pt=0  preci_type=Single  exp_width=8  frac_width=24  explicit_period=off  period=1  equ=P=C  opselect=C  inp2=PCIN>>17  opr=+  inp1=P  carry=CIN  dbl_ovrd=off  block_type=constant
  bit : xbsIndex_r4/Slice  nbits=1  boolean_output=off  mode=Lower Bit Location + Width  bit1=0  base1=MSB of Input  bit0=17  base0=LSB of Input  dbl_ovrd=off  block_type=slice
  force1 : xbsIndex_r4/Reinterpret  force_arith_type=on  arith_type="Signed  (2's comp)"  force_bin_pt=on  bin_pt=35  block_type=reinterpret
  force2 : xbsIndex_r4/Reinterpret  force_arith_type=off  arith_type="Signed  (2's comp)"  force_bin_pt=on  bin_pt=35  block_type=reinterpret
  tweak_op : xbsIndex_r4/Logical  logical_function=AND  inputs=2  en=off  latency=0  precision=Full  arith_type=Unsigned  n_bits=8  bin_pt=2  align_bp=on  dbl_ovrd=off  block_type=logical
  out : Outport
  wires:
  tweak_op/1 -> Concat/2
  Constant/1 -> tweak_op/2
  bit/1 -> tweak_op/1
  almost_half/1 -> force2/1
  in/1 -> Reinterpret/1, bit/1
  Concat/1 -> force1/1
  Reinterpret/1 -> Concat/1
  force1/1 -> adder/1
  force2/1 -> adder/2
  adder/1 -> out/1

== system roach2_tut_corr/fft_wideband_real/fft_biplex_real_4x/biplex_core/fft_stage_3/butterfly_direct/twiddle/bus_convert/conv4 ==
  note: (ones_bit & 1) -> round-to-even (ones_bit ^ 1) -> round-to-odd (sign_bit & 1)-> round-to-zero (sign_bit ^ 1) -> round-to-inf (X ~| 1) -> round half down (X | 1) -> round half up
  in : Inport
  Concat : xbsIndex_r4/Concat  num_inputs=2  dbl_ovrd=off  block_type=concat
  Constant : xbsIndex_r4/Constant  const=1  gui_display_data_type=Fixed-point  arith_type=Unsigned  n_bits=1  bin_pt=0  preci_type=Single  exp_width=8  frac_width=24  explicit_period=off  period=1  equ=P=C  opselect=C  inp2=PCIN>>17  opr=+  inp1=P  carry=CIN  dbl_ovrd=off  block_type=constant
  Reinterpret : xbsIndex_r4/Reinterpret  force_arith_type=on  arith_type=Unsigned  force_bin_pt=on  bin_pt=0  block_type=reinterpret
  adder : xbsIndex_r4/AddSub  mode=Addition  use_carryin=off  use_carryout=off  en=off  latency=1  precision=User Defined  arith_type="Signed  (2's comp)"  n_bits=19  bin_pt=17  quantization=Truncate  overflow=Wrap  dbl_ovrd=off  use_behavioral_HDL=off  hw_selection=Fabric  pipelined=on  use_rpm=on  block_type=addsub
  almost_half : xbsIndex_r4/Constant  const=131071  gui_display_data_type=Fixed-point  arith_type=Unsigned  n_bits=35  bin_pt=0  preci_type=Single  exp_width=8  frac_width=24  explicit_period=off  period=1  equ=P=C  opselect=C  inp2=PCIN>>17  opr=+  inp1=P  carry=CIN  dbl_ovrd=off  block_type=constant
  bit : xbsIndex_r4/Slice  nbits=1  boolean_output=off  mode=Lower Bit Location + Width  bit1=0  base1=MSB of Input  bit0=17  base0=LSB of Input  dbl_ovrd=off  block_type=slice
  force1 : xbsIndex_r4/Reinterpret  force_arith_type=on  arith_type="Signed  (2's comp)"  force_bin_pt=on  bin_pt=35  block_type=reinterpret
  force2 : xbsIndex_r4/Reinterpret  force_arith_type=off  arith_type="Signed  (2's comp)"  force_bin_pt=on  bin_pt=35  block_type=reinterpret
  tweak_op : xbsIndex_r4/Logical  logical_function=AND  inputs=2  en=off  latency=0  precision=Full  arith_type=Unsigned  n_bits=8  bin_pt=2  align_bp=on  dbl_ovrd=off  block_type=logical
  out : Outport
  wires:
  tweak_op/1 -> Concat/2
  Constant/1 -> tweak_op/2
  bit/1 -> tweak_op/1
  almost_half/1 -> force2/1
  in/1 -> Reinterpret/1, bit/1
  Concat/1 -> force1/1
  Reinterpret/1 -> Concat/1
  force1/1 -> adder/1
  force2/1 -> adder/2
  adder/1 -> out/1

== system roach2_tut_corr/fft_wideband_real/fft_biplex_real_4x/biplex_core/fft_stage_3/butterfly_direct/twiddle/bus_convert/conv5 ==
  note: (ones_bit & 1) -> round-to-even (ones_bit ^ 1) -> round-to-odd (sign_bit & 1)-> round-to-zero (sign_bit ^ 1) -> round-to-inf (X ~| 1) -> round half down (X | 1) -> round half up
  in : Inport
  Concat : xbsIndex_r4/Concat  num_inputs=2  dbl_ovrd=off  block_type=concat
  Constant : xbsIndex_r4/Constant  const=1  gui_display_data_type=Fixed-point  arith_type=Unsigned  n_bits=1  bin_pt=0  preci_type=Single  exp_width=8  frac_width=24  explicit_period=off  period=1  equ=P=C  opselect=C  inp2=PCIN>>17  opr=+  inp1=P  carry=CIN  dbl_ovrd=off  block_type=constant
  Reinterpret : xbsIndex_r4/Reinterpret  force_arith_type=on  arith_type=Unsigned  force_bin_pt=on  bin_pt=0  block_type=reinterpret
  adder : xbsIndex_r4/AddSub  mode=Addition  use_carryin=off  use_carryout=off  en=off  latency=1  precision=User Defined  arith_type="Signed  (2's comp)"  n_bits=19  bin_pt=17  quantization=Truncate  overflow=Wrap  dbl_ovrd=off  use_behavioral_HDL=off  hw_selection=Fabric  pipelined=on  use_rpm=on  block_type=addsub
  almost_half : xbsIndex_r4/Constant  const=131071  gui_display_data_type=Fixed-point  arith_type=Unsigned  n_bits=35  bin_pt=0  preci_type=Single  exp_width=8  frac_width=24  explicit_period=off  period=1  equ=P=C  opselect=C  inp2=PCIN>>17  opr=+  inp1=P  carry=CIN  dbl_ovrd=off  block_type=constant
  bit : xbsIndex_r4/Slice  nbits=1  boolean_output=off  mode=Lower Bit Location + Width  bit1=0  base1=MSB of Input  bit0=17  base0=LSB of Input  dbl_ovrd=off  block_type=slice
  force1 : xbsIndex_r4/Reinterpret  force_arith_type=on  arith_type="Signed  (2's comp)"  force_bin_pt=on  bin_pt=35  block_type=reinterpret
  force2 : xbsIndex_r4/Reinterpret  force_arith_type=off  arith_type="Signed  (2's comp)"  force_bin_pt=on  bin_pt=35  block_type=reinterpret
  tweak_op : xbsIndex_r4/Logical  logical_function=AND  inputs=2  en=off  latency=0  precision=Full  arith_type=Unsigned  n_bits=8  bin_pt=2  align_bp=on  dbl_ovrd=off  block_type=logical
  out : Outport
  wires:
  tweak_op/1 -> Concat/2
  Constant/1 -> tweak_op/2
  bit/1 -> tweak_op/1
  almost_half/1 -> force2/1
  in/1 -> Reinterpret/1, bit/1
  Concat/1 -> force1/1
  Reinterpret/1 -> Concat/1
  force1/1 -> adder/1
  force2/1 -> adder/2
  adder/1 -> out/1

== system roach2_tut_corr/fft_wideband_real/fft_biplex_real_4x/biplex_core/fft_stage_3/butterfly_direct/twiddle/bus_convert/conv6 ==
  note: (ones_bit & 1) -> round-to-even (ones_bit ^ 1) -> round-to-odd (sign_bit & 1)-> round-to-zero (sign_bit ^ 1) -> round-to-inf (X ~| 1) -> round half down (X | 1) -> round half up
  in : Inport
  Concat : xbsIndex_r4/Concat  num_inputs=2  dbl_ovrd=off  block_type=concat
  Constant : xbsIndex_r4/Constant  const=1  gui_display_data_type=Fixed-point  arith_type=Unsigned  n_bits=1  bin_pt=0  preci_type=Single  exp_width=8  frac_width=24  explicit_period=off  period=1  equ=P=C  opselect=C  inp2=PCIN>>17  opr=+  inp1=P  carry=CIN  dbl_ovrd=off  block_type=constant
  Reinterpret : xbsIndex_r4/Reinterpret  force_arith_type=on  arith_type=Unsigned  force_bin_pt=on  bin_pt=0  block_type=reinterpret
  adder : xbsIndex_r4/AddSub  mode=Addition  use_carryin=off  use_carryout=off  en=off  latency=1  precision=User Defined  arith_type="Signed  (2's comp)"  n_bits=19  bin_pt=17  quantization=Truncate  overflow=Wrap  dbl_ovrd=off  use_behavioral_HDL=off  hw_selection=Fabric  pipelined=on  use_rpm=on  block_type=addsub
  almost_half : xbsIndex_r4/Constant  const=131071  gui_display_data_type=Fixed-point  arith_type=Unsigned  n_bits=35  bin_pt=0  preci_type=Single  exp_width=8  frac_width=24  explicit_period=off  period=1  equ=P=C  opselect=C  inp2=PCIN>>17  opr=+  inp1=P  carry=CIN  dbl_ovrd=off  block_type=constant
  bit : xbsIndex_r4/Slice  nbits=1  boolean_output=off  mode=Lower Bit Location + Width  bit1=0  base1=MSB of Input  bit0=17  base0=LSB of Input  dbl_ovrd=off  block_type=slice
  force1 : xbsIndex_r4/Reinterpret  force_arith_type=on  arith_type="Signed  (2's comp)"  force_bin_pt=on  bin_pt=35  block_type=reinterpret
  force2 : xbsIndex_r4/Reinterpret  force_arith_type=off  arith_type="Signed  (2's comp)"  force_bin_pt=on  bin_pt=35  block_type=reinterpret
  tweak_op : xbsIndex_r4/Logical  logical_function=AND  inputs=2  en=off  latency=0  precision=Full  arith_type=Unsigned  n_bits=8  bin_pt=2  align_bp=on  dbl_ovrd=off  block_type=logical
  out : Outport
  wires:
  tweak_op/1 -> Concat/2
  Constant/1 -> tweak_op/2
  bit/1 -> tweak_op/1
  almost_half/1 -> force2/1
  in/1 -> Reinterpret/1, bit/1
  Concat/1 -> force1/1
  Reinterpret/1 -> Concat/1
  force1/1 -> adder/1
  force2/1 -> adder/2
  adder/1 -> out/1

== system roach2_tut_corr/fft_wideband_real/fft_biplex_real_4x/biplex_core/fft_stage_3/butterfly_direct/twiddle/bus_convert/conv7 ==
  note: (ones_bit & 1) -> round-to-even (ones_bit ^ 1) -> round-to-odd (sign_bit & 1)-> round-to-zero (sign_bit ^ 1) -> round-to-inf (X ~| 1) -> round half down (X | 1) -> round half up
  in : Inport
  Concat : xbsIndex_r4/Concat  num_inputs=2  dbl_ovrd=off  block_type=concat
  Constant : xbsIndex_r4/Constant  const=1  gui_display_data_type=Fixed-point  arith_type=Unsigned  n_bits=1  bin_pt=0  preci_type=Single  exp_width=8  frac_width=24  explicit_period=off  period=1  equ=P=C  opselect=C  inp2=PCIN>>17  opr=+  inp1=P  carry=CIN  dbl_ovrd=off  block_type=constant
  Reinterpret : xbsIndex_r4/Reinterpret  force_arith_type=on  arith_type=Unsigned  force_bin_pt=on  bin_pt=0  block_type=reinterpret
  adder : xbsIndex_r4/AddSub  mode=Addition  use_carryin=off  use_carryout=off  en=off  latency=1  precision=User Defined  arith_type="Signed  (2's comp)"  n_bits=19  bin_pt=17  quantization=Truncate  overflow=Wrap  dbl_ovrd=off  use_behavioral_HDL=off  hw_selection=Fabric  pipelined=on  use_rpm=on  block_type=addsub
  almost_half : xbsIndex_r4/Constant  const=131071  gui_display_data_type=Fixed-point  arith_type=Unsigned  n_bits=35  bin_pt=0  preci_type=Single  exp_width=8  frac_width=24  explicit_period=off  period=1  equ=P=C  opselect=C  inp2=PCIN>>17  opr=+  inp1=P  carry=CIN  dbl_ovrd=off  block_type=constant
  bit : xbsIndex_r4/Slice  nbits=1  boolean_output=off  mode=Lower Bit Location + Width  bit1=0  base1=MSB of Input  bit0=17  base0=LSB of Input  dbl_ovrd=off  block_type=slice
  force1 : xbsIndex_r4/Reinterpret  force_arith_type=on  arith_type="Signed  (2's comp)"  force_bin_pt=on  bin_pt=35  block_type=reinterpret
  force2 : xbsIndex_r4/Reinterpret  force_arith_type=off  arith_type="Signed  (2's comp)"  force_bin_pt=on  bin_pt=35  block_type=reinterpret
  tweak_op : xbsIndex_r4/Logical  logical_function=AND  inputs=2  en=off  latency=0  precision=Full  arith_type=Unsigned  n_bits=8  bin_pt=2  align_bp=on  dbl_ovrd=off  block_type=logical
  out : Outport
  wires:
  tweak_op/1 -> Concat/2
  Constant/1 -> tweak_op/2
  bit/1 -> tweak_op/1
  almost_half/1 -> force2/1
  in/1 -> Reinterpret/1, bit/1
  Concat/1 -> force1/1
  Reinterpret/1 -> Concat/1
  force1/1 -> adder/1
  force2/1 -> adder/2
  adder/1 -> out/1

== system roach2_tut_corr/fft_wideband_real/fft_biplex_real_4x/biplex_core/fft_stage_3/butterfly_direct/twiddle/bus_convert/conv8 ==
  note: (ones_bit & 1) -> round-to-even (ones_bit ^ 1) -> round-to-odd (sign_bit & 1)-> round-to-zero (sign_bit ^ 1) -> round-to-inf (X ~| 1) -> round half down (X | 1) -> round half up
  in : Inport
  Concat : xbsIndex_r4/Concat  num_inputs=2  dbl_ovrd=off  block_type=concat
  Constant : xbsIndex_r4/Constant  const=1  gui_display_data_type=Fixed-point  arith_type=Unsigned  n_bits=1  bin_pt=0  preci_type=Single  exp_width=8  frac_width=24  explicit_period=off  period=1  equ=P=C  opselect=C  inp2=PCIN>>17  opr=+  inp1=P  carry=CIN  dbl_ovrd=off  block_type=constant
  Reinterpret : xbsIndex_r4/Reinterpret  force_arith_type=on  arith_type=Unsigned  force_bin_pt=on  bin_pt=0  block_type=reinterpret
  adder : xbsIndex_r4/AddSub  mode=Addition  use_carryin=off  use_carryout=off  en=off  latency=1  precision=User Defined  arith_type="Signed  (2's comp)"  n_bits=19  bin_pt=17  quantization=Truncate  overflow=Wrap  dbl_ovrd=off  use_behavioral_HDL=off  hw_selection=Fabric  pipelined=on  use_rpm=on  block_type=addsub
  almost_half : xbsIndex_r4/Constant  const=131071  gui_display_data_type=Fixed-point  arith_type=Unsigned  n_bits=35  bin_pt=0  preci_type=Single  exp_width=8  frac_width=24  explicit_period=off  period=1  equ=P=C  opselect=C  inp2=PCIN>>17  opr=+  inp1=P  carry=CIN  dbl_ovrd=off  block_type=constant
  bit : xbsIndex_r4/Slice  nbits=1  boolean_output=off  mode=Lower Bit Location + Width  bit1=0  base1=MSB of Input  bit0=17  base0=LSB of Input  dbl_ovrd=off  block_type=slice
  force1 : xbsIndex_r4/Reinterpret  force_arith_type=on  arith_type="Signed  (2's comp)"  force_bin_pt=on  bin_pt=35  block_type=reinterpret
  force2 : xbsIndex_r4/Reinterpret  force_arith_type=off  arith_type="Signed  (2's comp)"  force_bin_pt=on  bin_pt=35  block_type=reinterpret
  tweak_op : xbsIndex_r4/Logical  logical_function=AND  inputs=2  en=off  latency=0  precision=Full  arith_type=Unsigned  n_bits=8  bin_pt=2  align_bp=on  dbl_ovrd=off  block_type=logical
  out : Outport
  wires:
  tweak_op/1 -> Concat/2
  Constant/1 -> tweak_op/2
  bit/1 -> tweak_op/1
  almost_half/1 -> force2/1
  in/1 -> Reinterpret/1, bit/1
  Concat/1 -> force1/1
  Reinterpret/1 -> Concat/1
  force1/1 -> adder/1
  force2/1 -> adder/2
  adder/1 -> out/1
